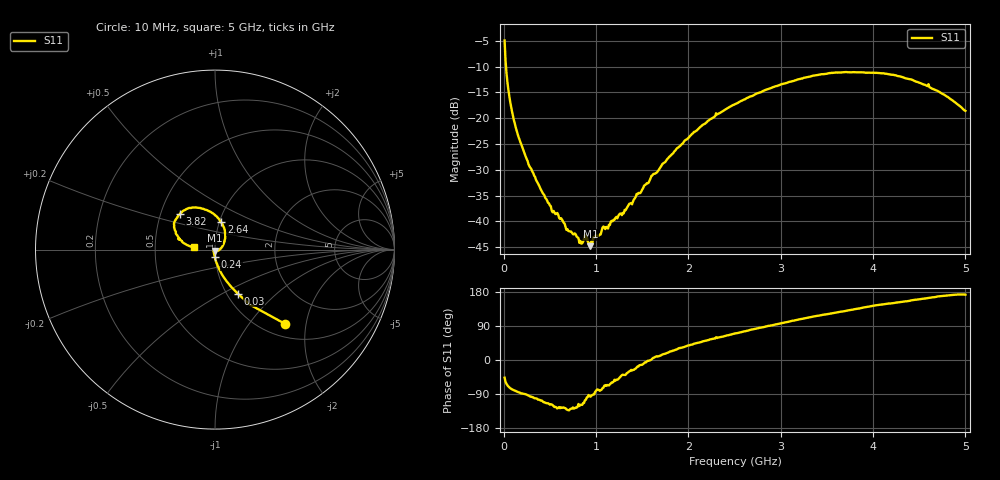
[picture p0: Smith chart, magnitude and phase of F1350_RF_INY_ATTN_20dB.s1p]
! S-parameters for RF_INY input IDT F1350 DPD Demodulator
! Date Measured:  2015-11-25  RGG
!  Port 1 = Pin 3 = RF_INY
! STATE: RF_INY selected, 20 dB attenuation (Gain = Gmax - 20 dB)
! RF Frequency:  10 MHz to 5000 MHz
! RF_INX, IF_I+, IF_I-, IF_Q+, and IF_Q- terminated
! 2300 MHz, 0 dBm signal applied to LO_IN
! Vcc = +5.00 Volts  Icc = approx 275 mA
! NOTES:  The device was measured on a custom printed circuit evaluation board with individual 50 ohm
!  microstrip lines to the RF and LO pins. The 50 ohm microstrip lines were de-embedded using reference
!  plane extensions
! Instrument Manufacturer:  Agilent Technologies
! Instrument Model:  E5071C
! Instrument Serial Number:  MY46419053
! Instrument Firmware Rev:  A.11.31
# HZ  S  RI R 50.00
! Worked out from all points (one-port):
!   500 points, 10 MHz to 5 GHz, reference 50 ohm
!   lowest |S11| = -44.8 dB at 940 MHz (marker M1), VSWR 1.01, Z = 49.9 - j0.57 ohm
!   |S11| at or under -10 dB: 25.06 MHz to end of sweep
!   S11 on the Smith chart (normalised r, x): 10 MHz: 1.25, -1.51; 30 MHz: 1.12, -0.60; 240 MHz: 1.00, -0.08; 2.64 GHz: 1.02, +0.32; 3.82 GHz: 0.63, +0.27; 5 GHz: 0.79, +0.03
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1e7  0.388 -0.4123
3e7  0.1268 -0.2452
4e7  0.0896 -0.2068
6e7  0.0509 -0.1571
1e8  0.021 -0.1035
1.6e8  0.00546 -0.0656
2.4e8  -0.000322 -0.0421
5.1e8  -0.00634 -0.0126
6.4e8  -0.00588 -0.00818
6.9e8  -0.00555 -0.00632
7.9e8  -0.00417 -0.00579
8.3e8  -0.00306 -0.0057
8.9e8  -0.00172 -0.00647
9.4e8  -0.000688 -0.00571
9.9e8  0.000755 -0.00723
1.26e9  0.00839 -0.0084
1.89e9  0.0449 0.0262
2.23e9  0.0568 0.0781
2.51e9  0.0461 0.1291
2.64e9  0.035 0.1536
3.13e9  -0.0545 0.2221
3.43e9  -0.1248 0.2346
3.76e9  -0.1859 0.2065
3.82e9  -0.1961 0.1973
4.13e9  -0.2274 0.1445
4.38e9  -0.2184 0.1003
4.7e9  -0.1793 0.0392
5e9  -0.1166 0.0156
